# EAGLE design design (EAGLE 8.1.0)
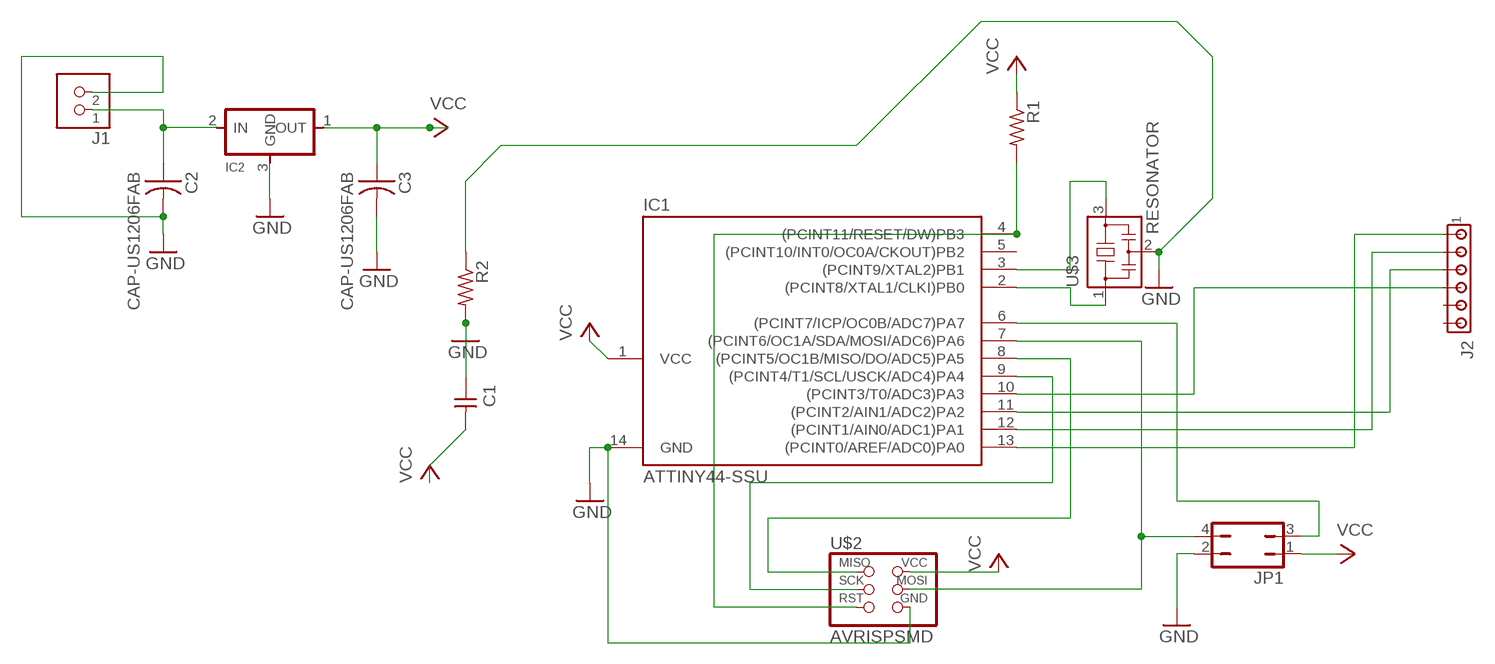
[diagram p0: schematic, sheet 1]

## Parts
C1  CAP-UNPOLARIZEDFAB  [C1206FAB]
C2  CAP-US1206FAB  [C1206FAB]
C3  CAP-US1206FAB  [C1206FAB]
IC1  ATTINY44-SSU  [SOIC14]
IC2  REGULATORSOT23  [SOT23]
J1  TERM-1X02-FABLAB  [ED555DS-2DS]
J2  MTA06-100  [10X06MTA]
JP1  JP2Q  [JP2Q]
R1  RES-US1206FAB  [R1206FAB]
R2  RES-US1206FAB  [R1206FAB]
U$2  AVRISPSMD  [2X03SMD]
U$3  RESONATOR  [EFOBM]

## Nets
GND: C1.1 C2.2 C3.2 IC1.14(GND) IC2.3(GND) J1.2 JP1.2 R2.1 R2.2 U$2.6(GND) U$3.2
N$1: IC1.2((PCINT8/XTAL1/CLKI)PB0) U$3.1
N$2: IC1.3((PCINT9/XTAL2)PB1) U$3.3
N$4: C2.1 IC2.2(IN) J1.1
N$5: IC1.7((PCINT6/OC1A/SDA/MOSI/ADC6)PA6) JP1.4 U$2.4(MOSI)
N$6: IC1.8((PCINT5/OC1B/MISO/DO/ADC5)PA5) U$2.1(MISO)
N$7: IC1.9((PCINT4/T1/SCL/USCK/ADC4)PA4) U$2.3(SCK)
N$8: IC1.13((PCINT0/AREF/ADC0)PA0) J2.1
N$9: IC1.6((PCINT7/ICP/OC0B/ADC7)PA7) JP1.3
N$11: IC1.12((PCINT1/AIN0/ADC1)PA1) J2.2
N$12: IC1.10((PCINT3/T0/ADC3)PA3) J2.4
N$13: IC1.11((PCINT2/AIN1/ADC2)PA2) J2.3
N$15: IC1.4((PCINT11/RESET/DW)PB3) R1.2 U$2.5(RST)
VCC: C1.2 C3.1 IC1.1(VCC) IC2.1(OUT) JP1.1 R1.1 U$2.2(VCC)
Unconnected: IC1.5((PCINT10/INT0/OC0A/CKOUT)PB2) J2.5 J2.6

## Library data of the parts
C1 = fab:CAP-UNPOLARIZED
C2 C3 = fab:CAP-US
IC1 = fab:ATTINY44
IC2 = fab:REGULATOR
J1 = fab:TERM-1X02: 3.5mm terminal block, 2 positions ED555-2DS as found in the fablab inventory.
J2 = con-amp:MTA06-100: AMP connector Connection corrected 2014-09-19
JP1 = jumper:JP2Q: JUMPER
R1 R2 = fab:RES-US: Resistor (US Symbol)
U$2 = fab:AVRISP
U$3 = fab:RESONATOR

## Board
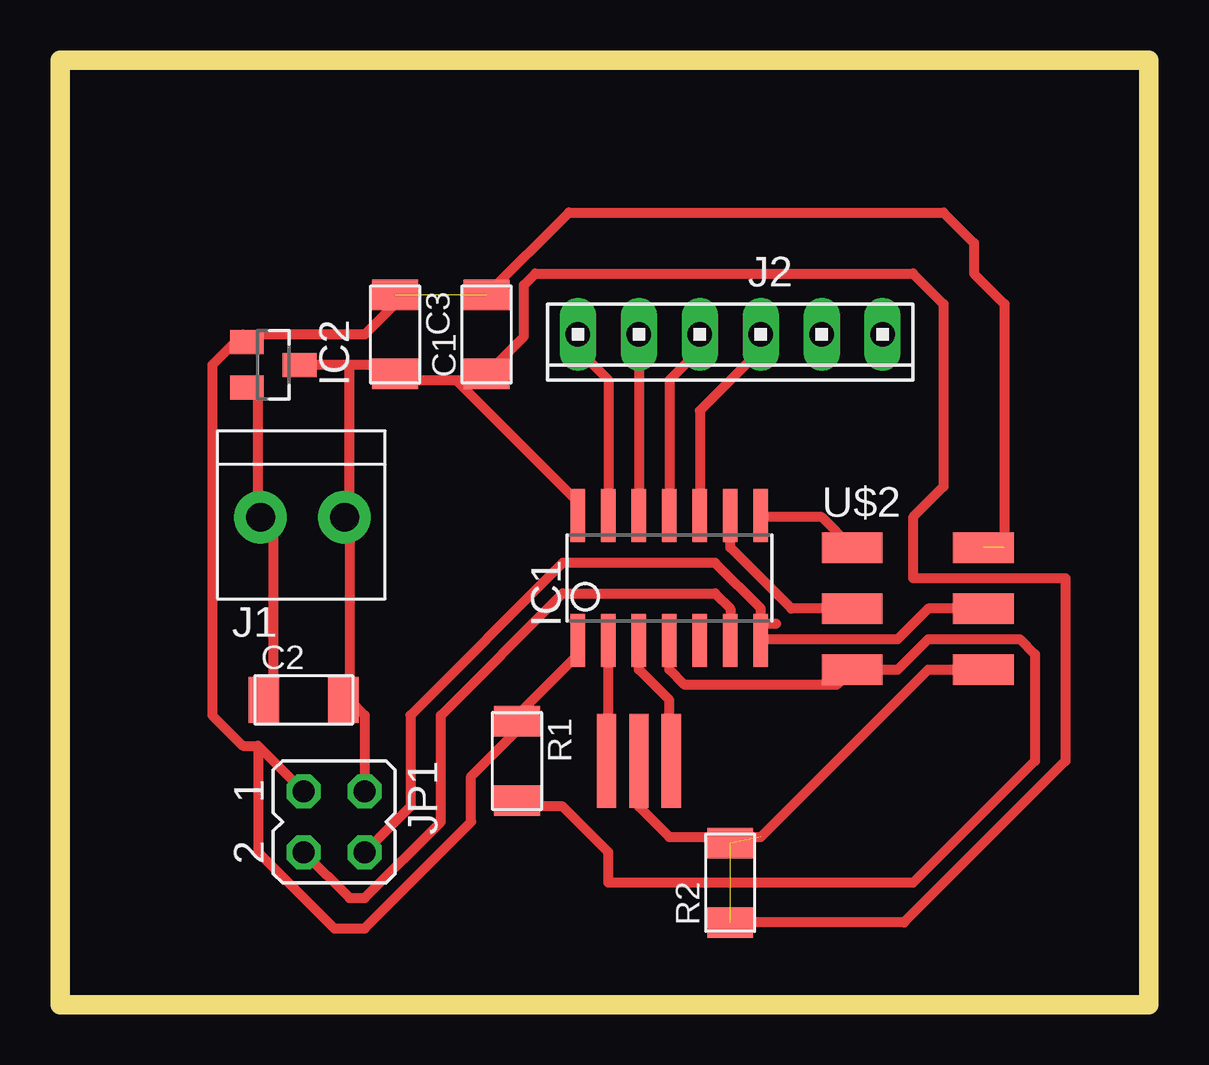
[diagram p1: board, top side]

Size 45.39 x 39.38 mm. Coordinates in mm from the lower left corner, seen from the top.
Outline: 0,0 45.39,0 45.39,39.36 0,39.38 0,0
Copper layers (1*16): Top 0.035mm / dielectric 1.5mm / Bottom 0.035mm
Design rules "default *": minimum track width 16mil, minimum drill 24mil, track to track 16mil, track to pad 16mil, pad to pad 16mil, via to via 16mil, smd to smd 8mil, copper to edge 40mil, drill to drill 8mil, minimum pad ring 10mil, minimum via ring 8mil, stop-mask expansion 4mil, vias tented up to drill 0mil, thermal gap 10mil

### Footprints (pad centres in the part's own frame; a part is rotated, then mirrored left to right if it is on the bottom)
C1206FAB = smd 1.27 x 1.905: 1 -1.651,0; 2 1.651,0
SOIC14 = smd 0.61 x 2.21: 1 -3.81,-2.603; 2 -2.54,-2.603; 3 -1.27,-2.603; 4 0,-2.603; 5 1.27,-2.603; 6 2.54,-2.603; 7 3.81,-2.603; 8 3.81,2.603; 9 2.54,2.603; 10 1.27,2.603; 11 0,2.603; 12 -1.27,2.603; 13 -2.54,2.603; 14 -3.81,2.603
SOT23 = smd 1 x 1.4: 1 -0.95,-1.1; 2 0.95,-1.1; 3 0,1.1
ED555DS-2DS = drill 1.2 pad 2.184: 1 1.8,0; 2 -1.7,0
10X06MTA = drill 1.016 long: 1 6.35,0; 2 3.81,0; 3 1.27,0; 4 -1.27,0; 5 -3.81,0; 6 -6.35,0
JP2Q = drill 0.914 octagon: 1 -1.27,-1.27; 2 -1.27,1.27; 3 1.27,-1.27; 4 1.27,1.27
R1206FAB = smd 1.27 x 1.905: 1 -1.651,0; 2 1.651,0
2X03SMD = smd 2.54 x 1.27: 1 -2.54,2.54; 2 2.92,2.54; 3 -2.54,0; 4 2.92,0; 5 -2.54,-2.54; 6 2.92,-2.54
EFOBM = smd 0.8 x 3.9: 1 -1.35,0; 2 0,0; 3 1.35,0

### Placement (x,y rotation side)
C1  17.78,27.94 90 top
C2  10.16,12.7 0 top
C3  13.97,27.94 270 top
IC1  25.4,17.78 0 top
IC2  8.89,26.67 270 top
J1  10.16,20.32 180 top
J2  27.94,27.94 180 top
JP1  11.43,7.62 270 top
R1  19.05,10.16 270 top
R2  27.94,5.08 90 top
U$2  35.56,16.51 0 top
U$3  24.13,10.16 0 top

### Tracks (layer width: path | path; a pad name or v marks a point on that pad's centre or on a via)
GND  (2 unrouted)
  Top 0.406: 12.07,26.67 13.97,26.67 C3.2 13.97,26.03 16.51,26.03 | 12.07,26.67 IC2.3 | 16.51,26.03 17.78,26.03 C1.1 19.34,27.85 19.34,30 19.82,30.48 35.56,30.48 36.83,29.21 36.83,21.59 35.56,20.32 35.56,17.78 41.91,17.78 41.91,10.16 35.18,3.43 R2.1 | 16.51,26.03 21.59,20.95 IC1.14 | 12.07,20.32 12.07,12.7 | JP1.2 12.7,12.06 12.07,12.7 | 12.07,12.7 C2.2 | 12.07,20.32 12.07,26.67 | 12.07,20.32 J1.2 | U$2.6 36.2,13.97 29.21,6.98 25.4,6.98 24.13,8.26 U$3.2
N$1
  Top 0.406: IC1.2 22.86,10.16 U$3.1
N$2
  Top 0.406: IC1.3 24.13,13.97 25.4,12.7 25.4,10.16 U$3.3
N$4
  Top 0.406: IC2.2 8.25,25.4 8.25,20.32 J1.1 8.89,20.32 8.89,12.7 C2.1
N$5
  Top 0.406: U$2.4 36.2,16.51 34.92,15.24 29.21,15.24 | JP1.4 14.61,8.26 14.61,12.06 20.96,18.41 27.31,18.41 29.21,16.51 29.21,15.88 | IC1.7 29.21,15.24 | 29.85,15.88 29.21,15.88 | 29.21,15.88 29.21,15.24
N$6
  Top 0.406: U$2.1 31.75,20.32 29.21,20.32 IC1.8
N$7
  Top 0.406: IC1.9 27.94,19.05 30.48,16.51 U$2.3
N$8
  Top 0.406: IC1.13 22.86,26.03 21.59,27.3 J2.1
N$9
  Top 0.406: IC1.6 27.94,16.51 27.31,17.15 20.96,17.15 15.88,12.06 15.88,7.62 12.7,4.45 12.07,4.45 JP1.3
N$11
  Top 0.406: J2.2 IC1.12
N$12
  Top 0.406: IC1.10 26.67,24.77 29.21,27.3 J2.4
N$13
  Top 0.406: IC1.11 25.4,26.03 26.67,27.3 J2.3
N$15
  Top 0.406: R1.2 19.05,8.26 20.96,8.26 22.86,6.35 22.86,5.08 35.56,5.08 40.64,10.16 40.64,14.6 40.01,15.24 36.2,15.24 34.92,13.97 U$2.5 32.39,13.34 26.04,13.34 25.4,13.97 IC1.4
VCC  (2 unrouted)
  Top 0.406: IC1.1 21.59,14.6 19.05,12.06 R1.1 19.05,11.43 17.14,9.52 17.14,7.62 12.7,3.17 11.43,3.17 8.25,6.35 8.25,10.8 | C3.1 13.97,29.21 12.7,27.94 8.25,27.94 IC2.1 7.62,27.94 6.35,26.67 6.35,12.06 7.62,10.8 8.25,10.8 | 8.25,10.8 JP1.1 | C1.2 21.21,33.02 36.83,33.02 38.1,31.75 38.1,30.48 39.37,29.21 39.37,19.05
